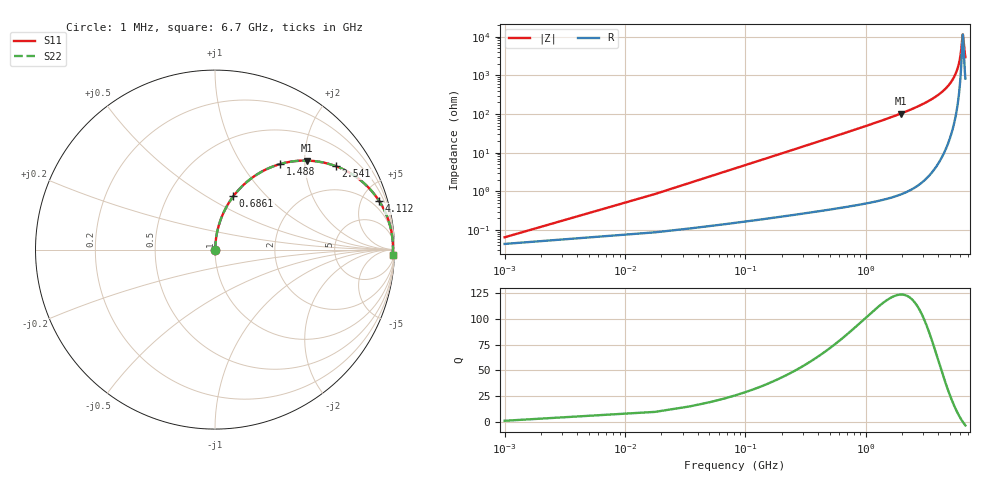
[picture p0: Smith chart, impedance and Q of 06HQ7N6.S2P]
! Coilcraft 0604HQ-7N6 Chip Inductor
! 15 August 2002
# MHZ S MA R 50
!Freq  MagS11  AngS11  MagS21  AngS21  MagS12  AngS12  MagS22  AngS22
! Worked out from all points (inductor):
!   402 points, 1 MHz to 6.7 GHz, reference 50 ohm
!   read as one part in series: L = 7.6 nH near 34.42 MHz
!   highest Q = 124 at 1.939 GHz (marker M1), where L = 8.37 nH
!   self-resonance near 6.368 GHz
!   S11 on the Smith chart (normalised r, x): 1 MHz: 1.00, +0.00; 686.1 MHz: 1.01, +0.66; 1.488 GHz: 1.01, +1.50; 2.541 GHz: 1.02, +2.88; 4.112 GHz: 1.12, +6.72; 6.7 GHz: 18, -57
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1  0.0006457 47.6  0.9996 -0.0  0.9996 -0.0  0.0006457 47.6
51.13  0.02441 85.6  0.9984 -1.4  0.9984 -1.4  0.02441 85.6
84.55  0.04032 85.5  0.9977 -2.3  0.9977 -2.3  0.04032 85.5
134.68  0.06412 84.7  0.9961 -3.7  0.9961 -3.7  0.06412 84.7
218.23  0.1036 82.8  0.9923 -5.9  0.9923 -5.9  0.1036 82.8
335.2  0.1581 79.9  0.9847 -9.1  0.9847 -9.1  0.1581 79.9
686.11  0.3135 71.0  0.9459 -18.3  0.9459 -18.3  0.3135 71.0
1120.57  0.4815 60.7  0.872 -28.8  0.872 -28.8  0.4815 60.7
1488.19  0.5984 52.8  0.7962 -36.8  0.7962 -36.8  0.5984 52.8
1939.36  0.7114 44.2  0.6971 -45.3  0.6971 -45.3  0.7114 44.2
2240.14  0.7704 39.1  0.6313 -50.4  0.6313 -50.4  0.7704 39.1
2540.92  0.8185 34.6  0.5675 -54.9  0.5675 -54.9  0.8185 34.6
3359.71  0.9079 24.1  0.4088 -65.2  0.4088 -65.2  0.9079 24.1
4111.66  0.9537 16.5  0.2838 -72.5  0.2838 -72.5  0.9537 16.5
4479.28  0.9679 13.2  0.2292 -75.4  0.2292 -75.4  0.9679 13.2
5114.26  0.9833 8.3  0.1438 -79.2  0.1438 -79.2  0.9833 8.3
5598.85  0.9892 4.9  0.08506 -80.3  0.08506 -80.3  0.9892 4.9
6050.02  0.9914 2.0  0.03519 -74.9  0.03519 -74.9  0.9914 2.0
6367.51  0.9914 0.1  0.008675 -6.4  0.008675 -6.4  0.9914 0.1
6417.64  0.9913 -0.2  0.009652 25.1  0.009652 25.1  0.9913 -0.2
6568.03  0.9908 -1.1  0.02122 63.7  0.02122 63.7  0.9908 -1.1
6700  0.9902 -1.8  0.03345 72.0  0.03345 72.0  0.9902 -1.8
